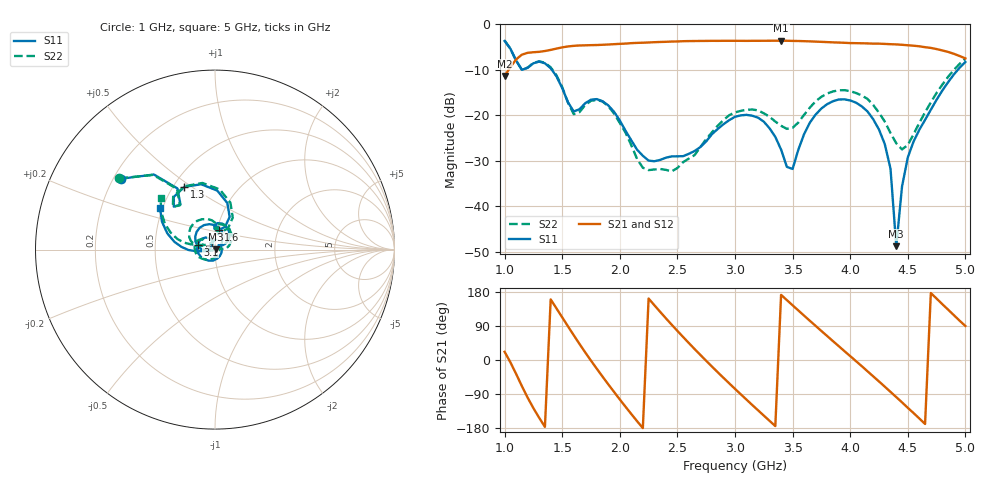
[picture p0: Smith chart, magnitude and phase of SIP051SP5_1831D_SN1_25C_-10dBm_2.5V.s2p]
# GHz  S  dB  R  50
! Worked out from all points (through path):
!   81 points, 1 GHz to 5 GHz, reference 50 ohm
!   highest |S21| = -3.61 dB at 3.4 GHz (marker M1); lowest = -11.4 dB at 1 GHz (marker M2)
!   lowest |S11| = -48.8 dB at 4.4 GHz (marker M3), VSWR 1.01, Z = 50.4 + j0.0855 ohm
!   |S11| at or under -10 dB: 1.149612 GHz to 1.151814 GHz (2.202 MHz wide, 0.191 % of centre); 1.409 GHz to 4.935 GHz (3.525 GHz wide, 111 % of centre)
!   |S22| runs from -32.4 to -3.6 dB; largest |S21 - S12| = 0.0041
!   S11 on the Smith chart (normalised r, x): 1 GHz: 0.23, +0.32; 1.3 GHz: 0.57, +0.47; 1.6 GHz: 1.02, +0.22; 3.1 GHz: 0.82, +0.05; 5 GHz: 0.48, +0.26
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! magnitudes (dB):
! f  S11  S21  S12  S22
! 1 GHz  -3.7  -11.4  -11.4  -3.6
! 1.15 GHz  -10.0  -6.7  -6.7  -10.0
! 1.3 GHz  -8.2  -6.1  -6.0  -8.1
! 1.45 GHz  -11.4  -5.3  -5.3  -11.2
! 1.6 GHz  -19.2  -4.7  -4.7  -19.8
! 1.7 GHz  -17.4  -4.6  -4.6  -17.7
! 1.9 GHz  -17.8  -4.4  -4.4  -18.0
! 2.2 GHz  -28.9  -4.0  -4.0  -31.6
! 2.35 GHz  -29.8  -3.9  -3.9  -31.8
! 2.65 GHz  -27.9  -3.7  -3.7  -28.8
! 3 GHz  -20.3  -3.6  -3.6  -19.4
! 3.1 GHz  -19.9  -3.6  -3.6  -18.8
! 3.4 GHz  -27.6  -3.6  -3.6  -22.3
! 3.5 GHz  -31.8  -3.7  -3.6  -22.8
! 3.7 GHz  -19.9  -3.8  -3.8  -16.9
! 4.1 GHz  -18.1  -4.2  -4.2  -15.7
! 4.25 GHz  -23.2  -4.3  -4.3  -19.5
! 4.35 GHz  -31.8  -4.4  -4.4  -23.9
! 4.4 GHz  -48.8  -4.4  -4.4  -26.2
! 4.45 GHz  -35.7  -4.5  -4.5  -27.5
! 4.55 GHz  -25.8  -4.7  -4.7  -24.2
! 5 GHz  -8.3  -7.5  -7.5  -7.6
